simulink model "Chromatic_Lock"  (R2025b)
settings: Solver=FixedStepDiscrete  StartTime=0.0  StopTime=inf  FixedStep=0.01  RelTol=1e-3  EnableMultiTasking=on
libraries: arduinolib x3
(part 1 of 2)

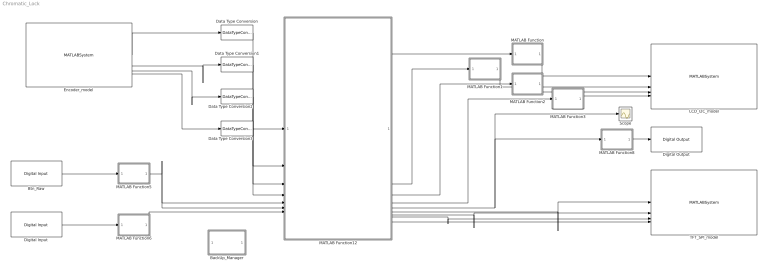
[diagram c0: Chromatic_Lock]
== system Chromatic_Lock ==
  BackUp_Manager : Subsystem  Commented=on
  Btn_Raw : arduinolib/Digital Input  pinNumber=6  mode=Default  Direction=input  SampleTime=0.1  blockPlatform=arduino
  Data Type Conversion{,1..3} (4 alike) : DataTypeConversion  OutDataTypeStr=double
  Digital Input : arduinolib/Digital Input  pinNumber=5  mode=Default  Direction=input  SampleTime=0.1  blockPlatform=arduino
  Digital Output : arduinolib/Digital Output  pinNumber=44  Direction=output  blockPlatform=arduino
  Encoder_model : MATLABSystem  System=Encoder  SampleTime=-1
  LCD_I2C_model : MATLABSystem  System=LCD_I2C  I2C_Address=uint8( 39 )  NumLines=uint8( 4 )  NumColumns=uint8( 20 )  SampleTime=-1
  MATLAB Function : MATLAB Function  TreatAsAtomicUnit=on
  MATLAB Function1 : MATLAB Function  TreatAsAtomicUnit=on
  MATLAB Function12 : MATLAB Function  TreatAsAtomicUnit=on
  MATLAB Function2 : MATLAB Function  TreatAsAtomicUnit=on
  MATLAB Function3 : MATLAB Function  TreatAsAtomicUnit=on
  MATLAB Function5 : MATLAB Function  TreatAsAtomicUnit=on
  MATLAB Function6 : MATLAB Function  TreatAsAtomicUnit=on
  MATLAB Function8 : MATLAB Function  TreatAsAtomicUnit=on
  Scope : Scope
  TFT_SPI_model : MATLABSystem  System=TFT_SPI  DC_Pin=uint8(10)  CS_Pin=uint8(8)  RESET_Pin=uint8(9)  BL_Pin=uint8(7)  SPI_Module=uint8(0)  Screen_Width=uint16(240)  Screen_Height=uint16(320)  Color_Mode=uint8(1)  SampleTime=-1
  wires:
  MATLAB Function12/3(L2) -> MATLAB Function1/1(str)
  MATLAB Function12/4(L3) -> MATLAB Function2/1(str)
  MATLAB Function12/5(L4) -> MATLAB Function3/1(str)
  MATLAB Function12/6(Tone_Event) -> MATLAB Function8/1(Tone_Event), Scope/1
  MATLAB Function12/2(L1) -> MATLAB Function/1(str)
  Btn_Raw/1 -> MATLAB Function5/1(btn_raw)
  MATLAB Function5/1(btn_out) -> MATLAB Function12/5(Match_Btn), MATLAB Function12/6(Select_Btn)
  Digital Input/1 -> MATLAB Function6/1(btn_raw)
  MATLAB Function6/1(btn_out) -> MATLAB Function12/7(Reset_Btn)
  MATLAB Function8/1(Tone_Freq) -> Digital Output/1
  MATLAB Function12/10(Mix_color) -> TFT_SPI_model/4
  MATLAB Function12/8(G_color) -> TFT_SPI_model/2
  MATLAB Function12/7(R_color) -> TFT_SPI_model/1
  MATLAB Function12/9(B_color) -> TFT_SPI_model/3
  Encoder_model/1 -> Data Type Conversion/1
  Encoder_model/2 -> Data Type Conversion1/1
  Encoder_model/3 -> Data Type Conversion2/1
  Encoder_model/4 -> Data Type Conversion3/1
  Data Type Conversion/1 -> MATLAB Function12/1(R_idx)
  Data Type Conversion1/1 -> MATLAB Function12/2(G_idx)
  MATLAB Function/1(out) -> LCD_I2C_model/1
  MATLAB Function1/1(out) -> LCD_I2C_model/2
  MATLAB Function2/1(out) -> LCD_I2C_model/3
  MATLAB Function3/1(out) -> LCD_I2C_model/4
  Data Type Conversion2/1 -> MATLAB Function12/3(B_idx)
  Data Type Conversion3/1 -> MATLAB Function12/4(Difficulty_Input)

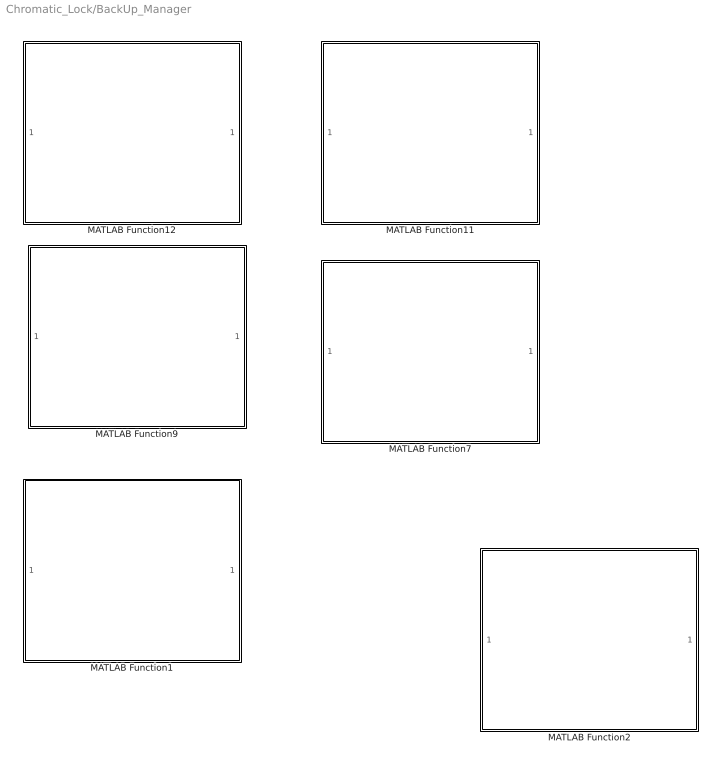
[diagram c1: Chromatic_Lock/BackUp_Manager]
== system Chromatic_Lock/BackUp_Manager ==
  MATLAB Function1 : MATLAB Function  Commented=on  TreatAsAtomicUnit=on
  MATLAB Function11 : MATLAB Function  Commented=on  TreatAsAtomicUnit=on
  MATLAB Function12 : MATLAB Function  Commented=on  TreatAsAtomicUnit=on
  MATLAB Function2 : MATLAB Function  Commented=on  TreatAsAtomicUnit=on
  MATLAB Function7 : MATLAB Function  Commented=on  TreatAsAtomicUnit=on
  MATLAB Function9 : MATLAB Function  Commented=on  TreatAsAtomicUnit=on

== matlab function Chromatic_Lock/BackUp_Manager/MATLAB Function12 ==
function [RGB, L1, L2, L3, L4, Buzzer] = ...
    Game_Manager(R_idx, G_idx, B_idx, Match_Btn, Select_Btn, Difficulty_Input, Reset_Btn)
%#codegen

%% ================= DATA TYPES =================
R_idx = uint8(R_idx);
G_idx = uint8(G_idx);
B_idx = uint8(B_idx);
Difficulty_Input = uint8(Difficulty_Input);

%% ============ PERSISTENT VARIABLES ============
persistent state puzzle_count puzzle_limit targets

if isempty(state)
    state = uint8(0);        % 0=Select Difficulty, 1=Play, 2=Complete
    puzzle_count = uint8(1);
    puzzle_limit = uint8(0);

    targets(1).R.idx = 2;
    targets(1).R.hints = ["Rot: Tomatenrot      ", "Rot: Ziegelrot       ", "Rot: Scharlach       "];
    targets(1).G.idx = 1;
    targets(1).G.hints = ["Gruen: Apfelgruen    ", "Gruen: Fruehlingsgruen", "Gruen: Moosgruen      "];
    targets(1).B.idx = 3;
    targets(1).B.hints = ["Blau: Azurblau       ", "Blau: EU-Blau        ", "Blau: Koenigsblau     "];

    targets(2).R.idx = 4;
    targets(2).R.hints = ["Rot: Kirschrot       ", "Rot: Rubinrot        ", "Rot: Purpur          "];
    targets(2).G.idx = 3;
    targets(2).G.hints = ["Gruen: Hoffnungsgruen", "Gruen: Smaragd       ", "Gruen: Tannengruen    "];
    targets(2).B.idx = 5;
    targets(2).B.hints = ["Blau: Marineblau     ", "Blau: Tiefsee        ", "Blau: Mitternacht    "];

    targets(3).R.idx = 6;
    targets(3).R.hints = ["Rot: Feuerrot        ", "Rot: Glutrot         ", "Rot: Vulkanrot       "];
    targets(3).G.idx = 1;
    targets(3).G.hints = ["Gruen: Apfelgruen    ", "Gruen: Limette       ", "Gruen: Farn          "];
    targets(3).B.idx = 3;
    targets(3).B.hints = ["Blau: Heraldik       ", "Blau: Stahlblau      ", "Blau: Polarblau      "];

    targets(4).R.idx = 3;
    targets(4).R.hints = ["Rot: Ziegelrot       ", "Rot: Terrakotta      ", "Rot: Ockerrot        "];
    targets(4).G.idx = 4;
    targets(4).G.hints = ["Gruen: Limettengruen ", "Gruen: Chartreuse    ", "Gruen: Neon          "];
    targets(4).B.idx = 2;
    targets(4).B.hints = ["Blau: Mittelmeer     ", "Blau: Kuestenblau    ", "Blau: Horizont       "];

    targets(5).R.idx = 5;
    targets(5).R.hints = ["Rot: Rosenrot        ", "Rot: Altrosa         ", "Rot: Pastellrot      "];
    targets(5).G.idx = 6;
    targets(5).G.hints = ["Gruen: Dschungelgruen", "Gruen: Tropengruen   ", "Gruen: Mangroven     "];
    targets(5).B.idx = 1;
    targets(5).B.hints = ["Blau: Eisblau        ", "Blau: EU-Blau        ", "Blau: Stahlblau      "];

    targets(6).R.idx = 1;
    targets(6).R.hints = ["Rot: Tomatenrot      ", "Rot: Bordeaux        ", "Rot: Burgunder       "];
    targets(6).G.idx = 2;
    targets(6).G.hints = ["Gruen: Irischgruen   ", "Gruen: Moosgruen     ", "Gruen: Waldgruen     "];
    targets(6).B.idx = 5;
    targets(6).B.hints = ["Blau: Marineblau     ", "Blau: Tiefsee        ", "Blau: Nachtblau       "];
end

%% ================= RESET ======================
if Reset_Btn
    state = uint8(0);
    puzzle_count = uint8(1);
    puzzle_limit = uint8(0);
end

%% ================= DEFAULT OUTPUTS ============
RGB = [0.2 0.2 0.2];
Buzzer = false;

L1 = uint8('                    ');
L2 = uint8('                    ');
L3 = uint8('                    ');
L4 = uint8('                    ');

palette = [1.0 0.8 0.6 0.4 0.2 0.1];

%% ================= FSM ========================
switch state

    % ========== STATE 0: SELECT DIFFICULTY ==========
    case 0
        L1 = uint8('-- SCHWIERIGKEIT -- ');
        L2 = uint8('1 L     2 M     3 S ');
        L3 = uint8('Waehlen & SEL drueck');
        L4 = uint8('                    ');

        if Select_Btn
            if Difficulty_Input == 1
                puzzle_limit = uint8(3);
            elseif Difficulty_Input == 2
                puzzle_limit = uint8(4);
            elseif Difficulty_Input == 3
                puzzle_limit = uint8(6);
            else
                puzzle_limit = uint8(0); % invalid selection
            end

            if puzzle_limit > 0
                puzzle_count = uint8(1);
                state = uint8(1);
            end
        end

        % ========== STATE 1: PLAY GAME ==========
    case 1
        tgtR = targets(puzzle_count).R.idx;
        tgtG = targets(puzzle_count).G.idx;
        tgtB = targets(puzzle_count).B.idx;

        % Live RGB mixing
        RGB = [
            palette(R_idx), ...
            palette(G_idx), ...
            palette(B_idx) ];

        % LCD Hint Layout (AS REQUESTED)
        L1 = uint8('Mische RGB nach Hint');
        L2 = uint8(targets(puzzle_count).R.hints(Difficulty_Input));
        L3 = uint8(targets(puzzle_count).G.hints(Difficulty_Input));
        L4 = uint8(targets(puzzle_count).B.hints(Difficulty_Input));

        % Match check (ONE PUZZLE AT A TIME)
        if Match_Btn && ...
                R_idx == tgtR && ...
                G_idx == tgtG && ...
                B_idx == tgtB

            if puzzle_count < puzzle_limit
                puzzle_count = puzzle_count + 1;
            else
                state = uint8(2);
            end
        end

        % ========== STATE 2: GAME COMPLETE ==========
    case 2
        RGB = [0 1 0];
        Buzzer = true;

        L1 = uint8('***   GLUECKWUNSCH  ');
        L2 = uint8('Alle Raetsel geloest');
        L3 = uint8('GEHEIMCODE:     4729');
        L4 = uint8('Reset fuer Neustart ');
end
end

%% ============ HINT FUNCTIONS ==================

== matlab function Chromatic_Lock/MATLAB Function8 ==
function Tone_Freq = Buzzer_Manager(Tone_Event)
%#codegen
% Tone_Event:
% 0 = none
% 1 = start tone
% 2 = success tone sequence
% 3 = failure tone

persistent state timer
if isempty(state)
    state = uint8(0);   % idle
    timer = uint16(0);
end

% Default output: no tone
Tone_Freq = uint16(0);

% Timing (sample time = 0.01s)
SHORT = uint16(10);    % 100 ms
LONG  = uint16(30);    % 300 ms
GAP   = uint16(10);    % 100 ms

% Frequencies
START_TONE   = uint16(600);
SUCCESS_1    = uint16(880);
SUCCESS_2    = uint16(1200);
FAIL_TONE    = uint16(200);

switch state

    % ============================================================
    % IDLE — wait for event
    % ============================================================
    case 0
        if Tone_Event == 1
            % START tone
            state = uint8(10);
            timer = SHORT;

        elseif Tone_Event == 2
            % SUCCESS tone sequence
            state = uint8(20);
            timer = SHORT;

        elseif Tone_Event == 3
            % FAILURE tone
            state = uint8(30);
            timer = LONG;
        end

    % ============================================================
    % START TONE (one short beep)
    % ============================================================
    case 10
        Tone_Freq = START_TONE;
        timer = timer - 1;
        if timer == 0
            state = uint8(0);
        end

    % ============================================================
    % SUCCESS TONE — first tone
    % ============================================================
    case 20
        Tone_Freq = SUCCESS_1;
        timer = timer - 1;
        if timer == 0
            state = uint8(21);
            timer = GAP;
        end

    % SUCCESS TONE — gap
    case 21
        Tone_Freq = uint16(0);
        timer = timer - 1;
        if timer == 0
            state = uint8(22);
            timer = SHORT;
        end

    % SUCCESS TONE — second tone
    case 22
        Tone_Freq = SUCCESS_2;
        timer = timer - 1;
        if timer == 0
            state = uint8(0);
        end

    % ============================================================
    % FAILURE TONE (one long low tone)
    % ============================================================
    case 30
        Tone_Freq = FAIL_TONE;
        timer = timer - 1;
        if timer == 0
            state = uint8(0);
        end
end

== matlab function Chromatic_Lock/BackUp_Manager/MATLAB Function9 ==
function [RGB, L1, L2, L3, L4, Tone_Event] = ...
    Game_Manager(R_idx, G_idx, B_idx, Match_Btn, Select_Btn, Difficulty_Input, Reset_Btn)
%#codegen

%% ================= DATA TYPES =================
R_idx = uint8(R_idx);
G_idx = uint8(G_idx);
B_idx = uint8(B_idx);
Difficulty_Input = uint8(Difficulty_Input);

% Clamp encoder indices to valid palette range
R_idx = max(uint8(1), min(uint8(6), R_idx));
G_idx = max(uint8(1), min(uint8(6), G_idx));
B_idx = max(uint8(1), min(uint8(6), B_idx));

% Clamp difficulty
Difficulty_Input = max(uint8(1), min(uint8(3), Difficulty_Input));

%% ============ PERSISTENT VARIABLES ============
persistent state puzzle_count puzzle_limit ...
    R_tgt G_tgt B_tgt ...
    R_hints G_hints B_hints

if isempty(state)
    state = uint8(0);  % welcome screen        % 0=Select Difficulty, 1=Play, 2=Complete
    puzzle_count = uint8(1);
    puzzle_limit = uint8(0);

    % --- Targets as numeric arrays (6 puzzles) ---
    R_tgt = zeros(6,1,'uint8');
    G_tgt = zeros(6,1,'uint8');
    B_tgt = zeros(6,1,'uint8');

    % --- Hints as cell arrays (6 puzzles x 3 difficulty levels) ---
    R_hints = cell(6,3);
    G_hints = cell(6,3);
    B_hints = cell(6,3);

    % ==================== PUZZLE 1 ====================
    R_tgt(1)      = uint8(2);
    R_hints{1,1}  = 'Rot: Tomatenrot      ';
    R_hints{1,2}  = 'Rot: Ziegelrot       ';
    R_hints{1,3}  = 'Rot: Scharlach       ';

    G_tgt(1)      = uint8(1);
    G_hints{1,1}  = 'Gruen: Apfelgruen    ';
    G_hints{1,2}  = 'Gruen: Fruehlingsgruen';
    G_hints{1,3}  = 'Gruen: Moosgruen      ';

    B_tgt(1)      = uint8(3);
    B_hints{1,1}  = 'Blau: Azurblau       ';
    B_hints{1,2}  = 'Blau: EU-Blau        ';
    B_hints{1,3}  = 'Blau: Koenigsblau     ';

    % ==================== PUZZLE 2 ====================
    R_tgt(2)      = uint8(4);
    R_hints{2,1}  = 'Rot: Kirschrot       ';
    R_hints{2,2}  = 'Rot: Rubinrot        ';
    R_hints{2,3}  = 'Rot: Purpur          ';

    G_tgt(2)      = uint8(3);
    G_hints{2,1}  = 'Gruen: Hoffnungsgruen';
    G_hints{2,2}  = 'Gruen: Smaragd       ';
    G_hints{2,3}  = 'Gruen: Tannengruen    ';

    B_tgt(2)      = uint8(5);
    B_hints{2,1}  = 'Blau: Marineblau     ';
    B_hints{2,2}  = 'Blau: Tiefsee        ';
    B_hints{2,3}  = 'Blau: Mitternacht    ';

    % ==================== PUZZLE 3 ====================
    R_tgt(3)      = uint8(6);
    R_hints{3,1}  = 'Rot: Feuerrot        ';
    R_hints{3,2}  = 'Rot: Glutrot         ';
    R_hints{3,3}  = 'Rot: Vulkanrot       ';

    G_tgt(3)      = uint8(1);
    G_hints{3,1}  = 'Gruen: Apfelgruen    ';
    G_hints{3,2}  = 'Gruen: Limette       ';
    G_hints{3,3}  = 'Gruen: Farn          ';

    B_tgt(3)      = uint8(3);
    B_hints{3,1}  = 'Blau: Heraldik       ';
    B_hints{3,2}  = 'Blau: Stahlblau      ';
    B_hints{3,3}  = 'Blau: Polarblau      ';

    % ==================== PUZZLE 4 ====================
    R_tgt(4)      = uint8(3);
    R_hints{4,1}  = 'Rot: Ziegelrot       ';
    R_hints{4,2}  = 'Rot: Terrakotta      ';
    R_hints{4,3}  = 'Rot: Ockerrot        ';

    G_tgt(4)      = uint8(4);
    G_hints{4,1}  = 'Gruen: Limettengruen ';
    G_hints{4,2}  = 'Gruen: Chartreuse    ';
    G_hints{4,3}  = 'Gruen: Neon          ';

    B_tgt(4)      = uint8(2);
    B_hints{4,1}  = 'Blau: Mittelmeer     ';
    B_hints{4,2}  = 'Blau: Kuestenblau    ';
    B_hints{4,3}  = 'Blau: Horizont       ';

    % ==================== PUZZLE 5 ====================
    R_tgt(5)      = uint8(5);
    R_hints{5,1}  = 'Rot: Rosenrot        ';
    R_hints{5,2}  = 'Rot: Altrosa         ';
    R_hints{5,3}  = 'Rot: Pastellrot      ';

    G_tgt(5)      = uint8(6);
    G_hints{5,1}  = 'Gruen: Dschungelgruen';
    G_hints{5,2}  = 'Gruen: Tropengruen   ';
    G_hints{5,3}  = 'Gruen: Mangroven     ';

    B_tgt(5)      = uint8(1);
    B_hints{5,1}  = 'Blau: Eisblau        ';
    B_hints{5,2}  = 'Blau: EU-Blau        ';
    B_hints{5,3}  = 'Blau: Stahlblau      ';

    % ==================== PUZZLE 6 ====================
    R_tgt(6)      = uint8(1);
    R_hints{6,1}  = 'Rot: Tomatenrot      ';
    R_hints{6,2}  = 'Rot: Bordeaux        ';
    R_hints{6,3}  = 'Rot: Burgunder       ';

    G_tgt(6)      = uint8(2);
    G_hints{6,1}  = 'Gruen: Irischgruen   ';
    G_hints{6,2}  = 'Gruen: Moosgruen     ';
    G_hints{6,3}  = 'Gruen: Waldgruen     ';

    B_tgt(6)      = uint8(5);
    B_hints{6,1}  = 'Blau: Marineblau     ';
    B_hints{6,2}  = 'Blau: Tiefsee        ';
    B_hints{6,3}  = 'Blau: Nachtblau      ';
end

%% ================= RESET ======================
if Reset_Btn
    state = uint8(0);   % welcome screen
    puzzle_count = uint8(1);
    puzzle_limit = uint8(0);
end

%% ================= DEFAULT OUTPUTS ============
RGB = [0.2 0.2 0.2];
Tone_Event = uint8(0);   % <--- NEW

L1 = uint8('                    ');
L2 = uint8('                    ');
L3 = uint8('                    ');
L4 = uint8('                    ');

palette = [1.0 0.8 0.6 0.4 0.2 0.1];

%% ================= FSM ========================
switch state

    % ========== STATE 0: WELCOME SCREEN ==========
    case 0
        L1 = uint8('   Chromatic Lock   ');
        L2 = uint8('       Bereit       ');
        L3 = uint8('                    ');
        L4 = uint8('Druecke zum Starten ');

        if Select_Btn
            state = uint8(1);   % go to difficulty selection
        end

        % ========== STATE 1: SELECT DIFFICULTY ==========
    case 1
        L1 = uint8('-- SCHWIERIGKEIT -- ');
        L2 = uint8('1 L     2 M     3 S ');
        L3 = uint8('Waehlen & SEL drueck');
        L4 = uint8('                    ');

        if Select_Btn
            if Difficulty_Input == 1
                puzzle_limit = uint8(3);
            elseif Difficulty_Input == 2
                puzzle_limit = uint8(4);
            elseif Difficulty_Input == 3
                puzzle_limit = uint8(6);
            else
                puzzle_limit = uint8(0);
            end

            if puzzle_limit > 0
                Tone_Event = uint8(1);
                puzzle_count = uint8(1);
                state = uint8(2);
            end
        end

        % ========== STATE 2: PLAY GAME ==========
    case 2
        tgtR = R_tgt(puzzle_count);
        tgtG = G_tgt(puzzle_count);
        tgtB = B_tgt(puzzle_count);

        RGB = [palette(R_idx), palette(G_idx), palette(B_idx)];

        diffIdx = Difficulty_Input;

        L1 = uint8('Mische RGB nach Hint');

        r_hint = char(R_hints{puzzle_count, diffIdx});
        g_hint = char(G_hints{puzzle_count, diffIdx});
        b_hint = char(B_hints{puzzle_count, diffIdx});

        if length(r_hint) < 20, r_hint = [r_hint, repmat(' ',1,20-length(r_hint))]; end
        if length(g_hint) < 20, g_hint = [g_hint, repmat(' ',1,20-length(g_hint))]; end
        if length(b_hint) < 20, b_hint = [b_hint, repmat(' ',1,20-length(b_hint))]; end

        L2 = zeros(1,20,'uint8');
        L3 = zeros(1,20,'uint8');
        L4 = zeros(1,20,'uint8');
        for i = 1:20
            L2(i) = uint8(r_hint(i));
            L3(i) = uint8(g_hint(i));
            L4(i) = uint8(b_hint(i));
        end

        if Match_Btn
            if R_idx == tgtR && G_idx == tgtG && B_idx == tgtB
                Tone_Event = uint8(2);
                if puzzle_count < puzzle_limit
                    puzzle_count = puzzle_count + 1;
                else
                    state = uint8(3);
                end
            else
                Tone_Event = uint8(3);
            end
        end

        % ========== STATE 3: GAME COMPLETE ==========
    case 3
        RGB = [0 1 0];
        Tone_Event = uint8(2);

        L1 = uint8('***   GLUECKWUNSCH  ');
        L2 = uint8('Alle Raetsel geloest');
        L3 = uint8('GEHEIMCODE:     4729');
        L4 = uint8('Reset fuer Neustart ');
end
end

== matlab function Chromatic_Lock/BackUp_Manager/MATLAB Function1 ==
function [RGB, L1, L2, L3, L4, Tone_Event] = ...
    Game_Manager(R_idx, G_idx, B_idx, Match_Btn, Select_Btn, Difficulty_Input, Reset_Btn)
%#codegen

%% ================= DATA TYPES =================
R_idx = uint8(R_idx);
G_idx = uint8(G_idx);
B_idx = uint8(B_idx);
Difficulty_Input = uint8(Difficulty_Input);

% Clamp encoder indices to valid palette range
R_idx = max(uint8(1), min(uint8(6), R_idx));
G_idx = max(uint8(1), min(uint8(6), G_idx));
B_idx = max(uint8(1), min(uint8(6), B_idx));

% Clamp difficulty
Difficulty_Input = max(uint8(1), min(uint8(3), Difficulty_Input));

%% ============ PERSISTENT VARIABLES ============
persistent state puzzle_count puzzle_limit ...
    R_tgt G_tgt B_tgt ...
    R_hints G_hints B_hints ...
    difficulty_level

if isempty(state)
    state = uint8(0);  % 0=Welcome, 1=Select Difficulty, 2=Play, 3=Complete
    puzzle_count = uint8(1);
    puzzle_limit = uint8(0);
    difficulty_level = uint8(0);

    % --- Targets as numeric arrays (6 puzzles) ---
    R_tgt = zeros(6,1,'uint8');
    G_tgt = zeros(6,1,'uint8');
    B_tgt = zeros(6,1,'uint8');

    % --- Hints as cell arrays (6 puzzles x 3 difficulty levels) ---
    R_hints = cell(6,3);
    G_hints = cell(6,3);
    B_hints = cell(6,3);

    % ==================== PUZZLES ====================
    % PUZZLE 1
    R_tgt(1) = 2; R_hints{1,1} = 'Rot: Tomatenrot      '; R_hints{1,2} = 'Rot: Ziegelrot       '; R_hints{1,3} = 'Rot: Scharlach       ';
    G_tgt(1) = 1; G_hints{1,1} = 'Gruen: Apfelgruen    '; G_hints{1,2} = 'Gruen: Fruehlingsgruen'; G_hints{1,3} = 'Gruen: Moosgruen      ';
    B_tgt(1) = 3; B_hints{1,1} = 'Blau: Azurblau       '; B_hints{1,2} = 'Blau: EU-Blau        '; B_hints{1,3} = 'Blau: Koenigsblau     ';

    % PUZZLE 2
    R_tgt(2) = 4; R_hints{2,1} = 'Rot: Kirschrot       '; R_hints{2,2} = 'Rot: Rubinrot        '; R_hints{2,3} = 'Rot: Purpur          ';
    G_tgt(2) = 3; G_hints{2,1} = 'Gruen: Hoffnungsgruen'; G_hints{2,2} = 'Gruen: Smaragd       '; G_hints{2,3} = 'Gruen: Tannengruen    ';
    B_tgt(2) = 5; B_hints{2,1} = 'Blau: Marineblau     '; B_hints{2,2} = 'Blau: Tiefsee        '; B_hints{2,3} = 'Blau: Mitternacht    ';

    % PUZZLE 3
    R_tgt(3) = 6; R_hints{3,1} = 'Rot: Feuerrot        '; R_hints{3,2} = 'Rot: Glutrot         '; R_hints{3,3} = 'Rot: Vulkanrot       ';
    G_tgt(3) = 1; G_hints{3,1} = 'Gruen: Apfelgruen    '; G_hints{3,2} = 'Gruen: Limette       '; G_hints{3,3} = 'Gruen: Farn          ';
    B_tgt(3) = 3; B_hints{3,1} = 'Blau: Heraldik       '; B_hints{3,2} = 'Blau: Stahlblau      '; B_hints{3,3} = 'Blau: Polarblau      ';

    % PUZZLE 4
    R_tgt(4) = 3; R_hints{4,1} = 'Rot: Ziegelrot       '; R_hints{4,2} = 'Rot: Terrakotta      '; R_hints{4,3} = 'Rot: Ockerrot        ';
    G_tgt(4) = 4; G_hints{4,1} = 'Gruen: Limettengruen '; G_hints{4,2} = 'Gruen: Chartreuse    '; G_hints{4,3} = 'Gruen: Neon          ';
    B_tgt(4) = 2; B_hints{4,1} = 'Blau: Mittelmeer     '; B_hints{4,2} = 'Blau: Kuestenblau    '; B_hints{4,3} = 'Blau: Horizont       ';

    % PUZZLE 5
    R_tgt(5) = 5; R_hints{5,1} = 'Rot: Rosenrot        '; R_hints{5,2} = 'Rot: Altrosa         '; R_hints{5,3} = 'Rot: Pastellrot      ';
    G_tgt(5) = 6; G_hints{5,1} = 'Gruen: Dschungelgruen'; G_hints{5,2} = 'Gruen: Tropengruen   '; G_hints{5,3} = 'Gruen: Mangroven     ';
    B_tgt(5) = 1; B_hints{5,1} = 'Blau: Eisblau        '; B_hints{5,2} = 'Blau: EU-Blau        '; B_hints{5,3} = 'Blau: Stahlblau      ';

    % PUZZLE 6
    R_tgt(6) = 1; R_hints{6,1} = 'Rot: Tomatenrot      '; R_hints{6,2} = 'Rot: Bordeaux        '; R_hints{6,3} = 'Rot: Burgunder       ';
    G_tgt(6) = 2; G_hints{6,1} = 'Gruen: Irischgruen   '; G_hints{6,2} = 'Gruen: Moosgruen     '; G_hints{6,3} = 'Gruen: Waldgruen     ';
    B_tgt(6) = 5; B_hints{6,1} = 'Blau: Marineblau     '; B_hints{6,2} = 'Blau: Tiefsee        '; B_hints{6,3} = 'Blau: Nachtblau      ';
end

%% ================= RESET ======================
if Reset_Btn
    state = uint8(0);   % welcome screen
    puzzle_count = uint8(1);
    puzzle_limit = uint8(0);
    difficulty_level = uint8(0);
end

%% ================= DEFAULT OUTPUTS ============
RGB = [0.2 0.2 0.2];
Tone_Event = uint8(0);

L1 = uint8('                    ');
L2 = uint8('                    ');
L3 = uint8('                    ');
L4 = uint8('                    ');

% --- Channel-specific palettes (0..1), 6 shades each ---
% These are placeholders: 6 distinct, ordered shades per channel.
% You can refine them later against real palettes / TFT look.
R_palette = [ ...
    1.00  0.00  0.00;  % bright red
    0.90  0.10  0.05;  % tomato-ish
    0.80  0.20  0.10;  % brick / tile
    0.70  0.05  0.10;  % cherry / ruby
    0.60  0.20  0.25;  % rose / pastel red
    0.45  0.00  0.05]; % dark / wine red

G_palette = [ ...
    0.00  1.00  0.00;  % bright green
    0.20  0.90  0.10;  % apple / fresh
    0.10  0.75  0.10;  % grass / hope
    0.60  0.90  0.10;  % lime / neon mix
    0.00  0.60  0.20;  % jungle
    0.00  0.40  0.05]; % dark forest

B_palette = [ ...
    0.30  0.60  1.00;  % azur / ice
    0.10  0.40  0.90;  % sea / coast
    0.05  0.20  0.70;  % heraldic blue
    0.00  0.10  0.50;  % marine
    0.00  0.05  0.30;  % deep / night
    0.05  0.05  0.20]; % midnight / very dark

%% ================= FSM ========================
switch state

    % ========== STATE 0: WELCOME SCREEN ==========
    case 0
        L1 = uint8('   Chromatic Lock   ');
        L2 = uint8('       Bereit       ');
        L3 = uint8('                    ');
        L4 = uint8('Druecke zum Starten ');

        if Select_Btn
            state = uint8(1);
        end

    % ========== STATE 1: SELECT DIFFICULTY ==========
    case 1
        L1 = uint8('-- SCHWIERIGKEIT -- ');

        % --- Visual feedback for selection ---
        if Difficulty_Input == 1
            L2 = uint8('> 1 LEICHT          ');
            L3 = uint8('  2 MITTEL          ');
            L4 = uint8('  3 SCHWER          ');
        elseif Difficulty_Input == 2
            L2 = uint8('  1 LEICHT          ');
            L3 = uint8('> 2 MITTEL          ');
            L4 = uint8('  3 SCHWER          ');
        elseif Difficulty_Input == 3
            L2 = uint8('  1 LEICHT          ');
            L3 = uint8('  2 MITTEL          ');
            L4 = uint8('> 3 SCHWER          ');
        end

        if Select_Btn
            % Freeze difficulty for this run
            difficulty_level = Difficulty_Input;

            if difficulty_level == 1
                puzzle_limit = uint8(3);
            elseif difficulty_level == 2
                puzzle_limit = uint8(4);
            elseif difficulty_level == 3
                puzzle_limit = uint8(6);
            else
                puzzle_limit = uint8(0);
            end

            if puzzle_limit > 0
                Tone_Event = uint8(1);
                puzzle_count = uint8(1);
                state = uint8(2);
            end
        end

    % ========== STATE 2: PLAY GAME ==========
    case 2
        tgtR = R_tgt(puzzle_count);
        tgtG = G_tgt(puzzle_count);
        tgtB = B_tgt(puzzle_count);

        % Build RGB from channel-specific palettes
        RGB = [ ...
            R_palette(R_idx,1), ...
            G_palette(G_idx,2), ...
            B_palette(B_idx,3)];

        % Safety: if difficulty_level somehow 0, default to 1
        if difficulty_level < 1 || difficulty_level > 3
            diffIdx = uint8(1);
        else
            diffIdx = difficulty_level;
        end

        L1 = uint8('Mische RGB nach Hint');

        % Hints: fixed per puzzle + difficulty, unaffected by scrolling
        r_hint = char(R_hints{puzzle_count, diffIdx});
        g_hint = char(G_hints{puzzle_count, diffIdx});
        b_hint = char(B_hints{puzzle_count, diffIdx});

        if length(r_hint) < 20, r_hint = [r_hint, repmat(' ',1,20-length(r_hint))]; end
        if length(g_hint) < 20, g_hint = [g_hint, repmat(' ',1,20-length(g_hint))]; end
        if length(b_hint) < 20, b_hint = [b_hint, repmat(' ',1,20-length(b_hint))]; end

        L2 = zeros(1,20,'uint8');
        L3 = zeros(1,20,'uint8');
        L4 = zeros(1,20,'uint8');
        for i = 1:20
            L2(i) = uint8(r_hint(i));
            L3(i) = uint8(g_hint(i));
            L4(i) = uint8(b_hint(i));
        end

        if Match_Btn
            if R_idx == tgtR && G_idx == tgtG && B_idx == tgtB
                Tone_Event = uint8(2);
                if puzzle_count < puzzle_limit
                    puzzle_count = puzzle_count + 1;
                else
                    state = uint8(3);
                end
            else
                Tone_Event = uint8(3);
            end
        end

    % ========== STATE 3: GAME COMPLETE ==========
    case 3
        RGB = [0 1 0];
        Tone_Event = uint8(2);

        L1 = uint8('***   GLUECKWUNSCH  ');
        L2 = uint8('Alle Raetsel geloest');
        L3 = uint8('GEHEIMCODE:     4729');
        L4 = uint8('Reset fuer Neustart ');
end
end

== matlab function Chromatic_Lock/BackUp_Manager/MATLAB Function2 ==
function [RGB, L1, L2, L3, L4, Tone_Event] = ...
    Game_Manager(R_idx, G_idx, B_idx, Match_Btn, Select_Btn, Difficulty_Input, Reset_Btn)
%#codegen

%% ================= DATA TYPES =================
R_idx = uint8(R_idx);
G_idx = uint8(G_idx);
B_idx = uint8(B_idx);
Difficulty_Input = uint8(Difficulty_Input);

% Clamp encoder indices to valid palette range
R_idx = max(uint8(1), min(uint8(6), R_idx));
G_idx = max(uint8(1), min(uint8(6), G_idx));
B_idx = max(uint8(1), min(uint8(6), B_idx));

% Clamp difficulty
Difficulty_Input = max(uint8(1), min(uint8(3), Difficulty_Input));

%% ============ PERSISTENT VARIABLES ============
persistent state puzzle_count puzzle_limit ...
    R_tgt G_tgt B_tgt ...
    R_hints G_hints B_hints ...
    difficulty_level

if isempty(state)
    state = uint8(0);  
    puzzle_count = uint8(1);
    puzzle_limit = uint8(0);
    difficulty_level = uint8(0);

    % --- Targets as numeric arrays (6 puzzles) ---
    R_tgt = zeros(6,1,'uint8');
    G_tgt = zeros(6,1,'uint8');
    B_tgt = zeros(6,1,'uint8');

    % --- Hints as cell arrays (6 puzzles x 3 difficulty levels) ---
    R_hints = cell(6,3);
    G_hints = cell(6,3);
    B_hints = cell(6,3);

    % ==================== PUZZLES ====================
    % PUZZLE 1
    R_tgt(1) = 2; 
    R_hints{1,1} = 'Rot: Tomatenrot     ';
    R_hints{1,2} = 'Rot: Ziegelrot      ';
    R_hints{1,3} = 'Rot: Scharlach      ';

    G_tgt(1) = 1; 
    G_hints{1,1} = 'Gruen: Apfelgruen   ';
    G_hints{1,2} = 'Gruen: Fruehlingsgrn';
    G_hints{1,3} = 'Gruen: Moosgruen    ';

    B_tgt(1) = 3; 
    B_hints{1,1} = 'Blau: Azurblau      ';
    B_hints{1,2} = 'Blau: EU-Blau       ';
    B_hints{1,3} = 'Blau: Koenigsblau   ';

    % PUZZLE 2
    R_tgt(2) = 4; 
    R_hints{2,1} = 'Rot: Kirschrot      ';
    R_hints{2,2} = 'Rot: Rubinrot       ';
    R_hints{2,3} = 'Rot: Purpur         ';

    G_tgt(2) = 3; 
    G_hints{2,1} = 'Gruen: Hoffnungsgrn ';
    G_hints{2,2} = 'Gruen: Smaragd      ';
    G_hints{2,3} = 'Gruen: Tannengruen  ';

    B_tgt(2) = 5; 
    B_hints{2,1} = 'Blau: Marineblau    ';
    B_hints{2,2} = 'Blau: Tiefsee       ';
    B_hints{2,3} = 'Blau: Mitternacht   ';

    % PUZZLE 3
    R_tgt(3) = 6; 
    R_hints{3,1} = 'Rot: Feuerrot       ';
    R_hints{3,2} = 'Rot: Glutrot        ';
    R_hints{3,3} = 'Rot: Vulkanrot      ';

    G_tgt(3) = 1; 
    G_hints{3,1} = 'Gruen: Apfelgruen   ';
    G_hints{3,2} = 'Gruen: Limette      ';
    G_hints{3,3} = 'Gruen: Farn         ';

    B_tgt(3) = 3; 
    B_hints{3,1} = 'Blau: Heraldik      ';
    B_hints{3,2} = 'Blau: Stahlblau     ';
    B_hints{3,3} = 'Blau: Polarblau     ';

    % PUZZLE 4
    R_tgt(4) = 3; 
    R_hints{4,1} = 'Rot: Ziegelrot      ';
    R_hints{4,2} = 'Rot: Terrakotta     ';
    R_hints{4,3} = 'Rot: Ockerrot       ';

    G_tgt(4) = 4; 
    G_hints{4,1} = 'Gruen: Limettengrn  ';
    G_hints{4,2} = 'Gruen: Chartreuse   ';
    G_hints{4,3} = 'Gruen: Neon         ';

    B_tgt(4) = 2; 
    B_hints{4,1} = 'Blau: Mittelmeer    ';
    B_hints{4,2} = 'Blau: Kuestenblau   ';
    B_hints{4,3} = 'Blau: Horizont      ';

    % PUZZLE 5
    R_tgt(5) = 5; 
    R_hints{5,1} = 'Rot: Rosenrot       ';
    R_hints{5,2} = 'Rot: Altrosa        ';
    R_hints{5,3} = 'Rot: Pastellrot     ';

    G_tgt(5) = 6; 
    G_hints{5,1} = 'Gruen: Dschungelgrn ';
    G_hints{5,2} = 'Gruen: Tropengruen  ';
    G_hints{5,3} = 'Gruen: Mangroven    ';

    B_tgt(5) = 1; 
    B_hints{5,1} = 'Blau: Eisblau       ';
    B_hints{5,2} = 'Blau: EU-Blau       ';
    B_hints{5,3} = 'Blau: Stahlblau     ';

    % PUZZLE 6
    R_tgt(6) = 1; 
    R_hints{6,1} = 'Rot: Tomatenrot     ';
    R_hints{6,2} = 'Rot: Bordeaux       ';
    R_hints{6,3} = 'Rot: Burgunder      ';

    G_tgt(6) = 2; 
    G_hints{6,1} = 'Gruen: Irischgruen  ';
    G_hints{6,2} = 'Gruen: Moosgruen    ';
    G_hints{6,3} = 'Gruen: Waldgruen    ';

    B_tgt(6) = 5; 
    B_hints{6,1} = 'Blau: Marineblau    ';
    B_hints{6,2} = 'Blau: Tiefsee       ';
    B_hints{6,3} = 'Blau: Nachtblau     ';
end

%% ================= RESET ======================
if Reset_Btn
    state = uint8(0);
    puzzle_count = uint8(1);
    puzzle_limit = uint8(0);
    difficulty_level = uint8(0);
end

%% ================= DEFAULT OUTPUTS ============
RGB = [0.2 0.2 0.2];
Tone_Event = uint8(0);

L1 = uint8('                    ');
L2 = uint8('                    ');
L3 = uint8('                    ');
L4 = uint8('                    ');

%% ================= REAL COLOR PALETTES =================
R_palette = [ ...
    1.00 0.10 0.10;
    0.95 0.25 0.15;
    0.80 0.30 0.20;
    0.70 0.10 0.15;
    0.85 0.55 0.60;
    0.45 0.00 0.05];

G_palette = [ ...
    0.10 1.00 0.10;
    0.30 0.90 0.20;
    0.10 0.75 0.10;
    0.70 1.00 0.10;
    0.00 0.60 0.20;
    0.00 0.40 0.05];

B_palette = [ ...
    0.30 0.60 1.00;
    0.10 0.40 0.90;
    0.05 0.20 0.70;
    0.00 0.10 0.50;
    0.00 0.05 0.30;
    0.05 0.05 0.20];

%% ================= FSM ========================
switch state

    % WELCOME
    case 0
        RGB = [0.2 0.2 0.2];
        L1 = uint8('   Chromatic Lock   ');
        L2 = uint8('       Bereit       ');
        L3 = uint8('                    ');
        L4 = uint8('Druecke zum Starten ');

        if Select_Btn
            state = uint8(1);
        end

    % SELECT DIFFICULTY
    case 1
        RGB = [0.2 0.2 0.2];
        L1 = uint8('-- SCHWIERIGKEIT -- ');

        if Difficulty_Input == 1
            L2 = uint8('> 1 LEICHT          ');
            L3 = uint8('  2 MITTEL          ');
            L4 = uint8('  3 SCHWER          ');
        elseif Difficulty_Input == 2
            L2 = uint8('  1 LEICHT          ');
            L3 = uint8('> 2 MITTEL          ');
            L4 = uint8('  3 SCHWER          ');
        elseif Difficulty_Input == 3
            L2 = uint8('  1 LEICHT          ');
            L3 = uint8('  2 MITTEL          ');
            L4 = uint8('> 3 SCHWER          ');
        end

        if Select_Btn
            difficulty_level = Difficulty_Input;

            if difficulty_level == 1
                puzzle_limit = uint8(3);
            elseif difficulty_level == 2
                puzzle_limit = uint8(4);
            elseif difficulty_level == 3
                puzzle_limit = uint8(6);
            end

            Tone_Event = uint8(1);
            puzzle_count = uint8(1);
            state = uint8(2);
        end

    % PLAY GAME
    case 2
        tgtR = R_tgt(puzzle_count);
        tgtG = G_tgt(puzzle_count);
        tgtB = B_tgt(puzzle_count);

        RGB = [ ...
            R_palette(R_idx,1), ...
            G_palette(G_idx,2), ...
            B_palette(B_idx,3)];

        diffIdx = difficulty_level;
        if diffIdx < 1 || diffIdx > 3
            diffIdx = uint8(1);
        end

        L1 = uint8('Mische RGB nach Hint');

        r_hint = char(R_hints{puzzle_count, diffIdx});
        g_hint = char(G_hints{puzzle_count, diffIdx});
        b_hint = char(B_hints{puzzle_count, diffIdx});

        % Safety: enforce 20 chars
        if length(r_hint) > 20, r_hint = r_hint(1:20); end
        if length(g_hint) > 20, g_hint = g_hint(1:20); end
        if length(b_hint) > 20, b_hint = b_hint(1:20); end

        if length(r_hint) < 20, r_hint = [r_hint, repmat(' ',1,20-length(r_hint))]; end
        if length(g_hint) < 20, g_hint = [g_hint, repmat(' ',1,20-length(g_hint))]; end
        if length(b_hint) < 20, b_hint = [b_hint, repmat(' ',1,20-length(b_hint))]; end

        L2 = uint8(r_hint);
        L3 = uint8(g_hint);
        L4 = uint8(b_hint);

        if Match_Btn
            if R_idx == tgtR && G_idx == tgtG && B_idx == tgtB
                Tone_Event = uint8(2);
                if puzzle_count < puzzle_limit
                    puzzle_count = puzzle_count + 1;
                else
                    state = uint8(3);
                end
            else
                Tone_Event = uint8(3);
            end
        end

    % COMPLETE
    case 3
        RGB = [0 1 0];
        Tone_Event = uint8(2);

        L1 = uint8('***   GLUECKWUNSCH  ');
        L2 = uint8('Alle Raetsel geloest');
        L3 = uint8('GEHEIMCODE:     4729');
        L4 = uint8('Reset fuer Neustart ');

    % SAFETY FALLBACK (for any unexpected state)
    otherwise
        RGB = [0.2 0.2 0.2];
        Tone_Event = uint8(0);
        L1 = uint8(' UNGUELTIGER ZUSTAND');
        L2 = uint8('                    ');
        L3 = uint8('                    ');
        L4 = uint8('                    ');
        state = uint8(0);
end
end

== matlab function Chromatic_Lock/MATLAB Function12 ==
function [RGB, L1, L2, L3, L4, Tone_Event, ...
    R_color, G_color, B_color, Mix_color] = ...
    Game_Manager(R_idx, G_idx, B_idx, Difficulty_Input, ...
    Match_Btn, Select_Btn, Reset_Btn)
%#codegen

%% ================= INPUTS =================
R_idx = uint8(max(1,min(6,R_idx)));
G_idx = uint8(max(1,min(6,G_idx)));
B_idx = uint8(max(1,min(6,B_idx)));
Difficulty_Input = uint8(max(1,min(3,Difficulty_Input)));

%% ================= PERSISTENT =================
persistent state puzzle total_puzzles
persistent tgtR tgtG tgtB
persistent HintR HintG HintB

if isempty(state)
    state = uint8(0);
    puzzle = uint8(1);
    total_puzzles = uint8(3);

    % --- TARGETS (6 MAX) ---
    tgtR = uint8([2 4 6 3 5 1]);
    tgtG = uint8([1 3 1 4 6 2]);
    tgtB = uint8([3 5 3 2 1 5]);

    % --- HINTS (puzzle, difficulty, 20 chars) ---
    HintR = uint8(zeros(6,3,20));
    HintG = uint8(zeros(6,3,20));
    HintB = uint8(zeros(6,3,20));

    HintR(1,1,:) = uint8('Rot: Hell           ');
    HintR(1,2,:) = uint8('Rot: Mittel         ');
    HintR(1,3,:) = uint8('Rot: Dunkel         ');

    HintG(1,1,:) = uint8('Gruen: Frisch       ');
    HintG(1,2,:) = uint8('Gruen: Wald         ');
    HintG(1,3,:) = uint8('Gruen: Moos         ');

    HintB(1,1,:) = uint8('Blau: Himmel        ');
    HintB(1,2,:) = uint8('Blau: Meer          ');
    HintB(1,3,:) = uint8('Blau: Nacht         ');
end

%% ================= RESET =================
if Reset_Btn
    state = uint8(0);
    puzzle = uint8(1);
    total_puzzles = uint8(3);
end

%% ================= DEFAULT OUTPUT =================
RGB = [0.2 0.2 0.2];
Tone_Event = uint8(0);

L1 = uint8('                    ');
L2 = L1; L3 = L1; L4 = L1;

% TFT COLORS (LIVE)
R_color = single(R_idx) / 6;
G_color = single(G_idx) / 6;
B_color = single(B_idx) / 6;
Mix_color = (R_color + G_color + B_color) / 3;

%% ================= FSM =================
switch state

    % ---------- STATE 0 : WELCOME ----------
    case 0
        L1 = uint8('  CHROMATIC LOCK    ');
        L2 = uint8('                    ');
        L4 = uint8('Druecke Start       ');

        if Select_Btn
            state = uint8(1);
        end

        % ---------- STATE 1 : DIFFICULTY ----------
    case 1
        L1 = uint8('-- SCHWIERIGKEIT -- ');

        if Difficulty_Input == 1
            L2 = uint8('> LEICHT  (3)       ');
            L3 = uint8('  MITTEL  (4)       ');
            L4 = uint8('  SCHWER  (6)       ');
        elseif Difficulty_Input == 2
            L2 = uint8('  LEICHT  (3)       ');
            L3 = uint8('> MITTEL  (4)       ');
            L4 = uint8('  SCHWER  (6)       ');
        else
            L2 = uint8('  LEICHT  (3)       ');
            L3 = uint8('  MITTEL  (4)       ');
            L4 = uint8('> SCHWER  (6)       ');
        end

        if Select_Btn
            if Difficulty_Input == 1
                total_puzzles = uint8(3);
            elseif Difficulty_Input == 2
                total_puzzles = uint8(4);
            else
                total_puzzles = uint8(6);
            end
            puzzle = uint8(1);
            state = uint8(2);
        end

        % ---------- STATE 2 : PLAY ----------
    case 2
        L1 = uint8('Mische RGB nach Hint');

        L2 = reshape(HintR(puzzle,Difficulty_Input,:),1,20);
        L3 = reshape(HintG(puzzle,Difficulty_Input,:),1,20);
        L4 = reshape(HintB(puzzle,Difficulty_Input,:),1,20);

        if Match_Btn
            if R_idx == tgtR(puzzle) && ...
                    G_idx == tgtG(puzzle) && ...
                    B_idx == tgtB(puzzle)

                Tone_Event = uint8(1); % success
                puzzle = puzzle + 1;

                if puzzle > total_puzzles
                    state = uint8(3);
                end
            else
                Tone_Event = uint8(2); % error
            end
        end

        % ---------- STATE 3 : WIN ----------
    case 3
        RGB = [0 1 0];
        L1 = uint8('*** GEWONNEN ***    ');
        L2 = uint8('Alle Raetsel geloest');
        L3 = uint8('CODE: 4729          ');
        L4 = uint8('Reset zum Neustart  ');
end

end

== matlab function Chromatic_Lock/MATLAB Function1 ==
function out = pad20(str)
%#codegen
% Ensures fixed 20-char uint8 row vector for LCD

% Convert to char safely
str = char(str(:).');   % force row vector

n = length(str);

if n >= 20
    out = uint8(str(1:20));
else
    out = uint8([str repmat(' ', 1, 20-n)]);
end
end

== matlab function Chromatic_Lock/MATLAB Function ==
function out = pad20(str)
%#codegen
% Ensures fixed 20-char uint8 row vector for LCD

% Convert to char safely
str = char(str(:).');   % force row vector

n = length(str);

if n >= 20
    out = uint8(str(1:20));
else
    out = uint8([str repmat(' ', 1, 20-n)]);
end
end

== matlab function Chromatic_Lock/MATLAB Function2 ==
function out = pad20(str)
%#codegen
% Ensures fixed 20-char uint8 row vector for LCD

% Convert to char safely
str = char(str(:).');   % force row vector

n = length(str);

if n >= 20
    out = uint8(str(1:20));
else
    out = uint8([str repmat(' ', 1, 20-n)]);
end
end

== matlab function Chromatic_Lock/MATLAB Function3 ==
function out = pad20(str)
%#codegen
% Ensures fixed 20-char uint8 row vector for LCD

% Convert to char safely
str = char(str(:).');   % force row vector

n = length(str);

if n >= 20
    out = uint8(str(1:20));
else
    out = uint8([str repmat(' ', 1, 20-n)]);
end
end

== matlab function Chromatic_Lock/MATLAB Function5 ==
function btn_out = DebounceButton(btn_raw)
%#codegen
% btn_raw: 1 = released (pullup), 0 = pressed
% btn_out: 1 = single clean press event

persistent stable_state counter
if isempty(stable_state)
    stable_state = uint8(1);   % idle high
    counter = uint8(0);
end

btn_out = uint8(0);

% number of consecutive samples required
DEBOUNCE_CNT = uint8(3);   % adjust if needed

if btn_raw == stable_state
    counter = uint8(0);
else
    counter = counter + 1;
    if counter >= DEBOUNCE_CNT
        % state change confirmed
        stable_state = uint8(btn_raw);
        counter = uint8(0);

        % detect falling edge AFTER debounce
        if stable_state == 0
            btn_out = uint8(1);
        end
    end
end
end

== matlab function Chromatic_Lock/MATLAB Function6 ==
function btn_out = DebounceButton(btn_raw)
%#codegen
% btn_raw: 1 = released (pullup), 0 = pressed
% btn_out: 1 = single clean press event

persistent stable_state counter
if isempty(stable_state)
    stable_state = uint8(1);   % idle high
    counter = uint8(0);
end

btn_out = uint8(0);

% number of consecutive samples required
DEBOUNCE_CNT = uint8(3);   % adjust if needed

if btn_raw == stable_state
    counter = uint8(0);
else
    counter = counter + 1;
    if counter >= DEBOUNCE_CNT
        % state change confirmed
        stable_state = uint8(btn_raw);
        counter = uint8(0);

        % detect falling edge AFTER debounce
        if stable_state == 0
            btn_out = uint8(1);
        end
    end
end
end
